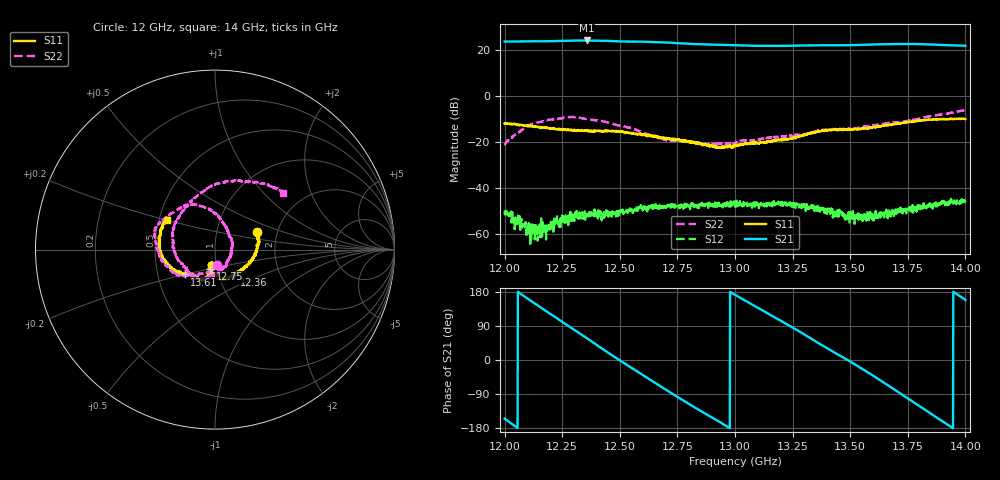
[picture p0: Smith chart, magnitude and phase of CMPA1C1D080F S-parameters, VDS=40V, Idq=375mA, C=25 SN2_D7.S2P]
!Keysight Technologies,E5071C,MY46632380,B.14.03
!Date: Thu Nov 05 05:05:17 2020
!Data & Calibration Information:
!Freq	S11:SOLT2(ON)	S21:SOLT2(ON)	S12:SOLT2(ON)	S22:SOLT2(ON)
!PortZ  Port1:50+j0  Port2:50+j0
!Above PortZ is port z conversion or system Z0 setting when saving the data.
!When reading, reference impedance value at option line is always used.
# Hz S dB R 50
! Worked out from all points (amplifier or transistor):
!   1601 points, 12 GHz to 14 GHz, reference 50 ohm
!   highest |S21| = 24.2 dB at 12.36 GHz (marker M1)
!   |S21| within 3 dB of that: start of sweep to end of sweep
!   unconditionally stable (mu >= 1): start of sweep to end of sweep
!   at 12.33 GHz: K = 11.18, MAG = 24.8 dB, |S12| = -52.4 dB
!   at 13 GHz: K = 8.22, MAG = 22.2 dB, |S12| = -46.5 dB
!   at 14 GHz: K = 5.41, MAG = 23.5 dB, |S12| = -45.8 dB
!   S11 on the Smith chart (normalised r, x): 12 GHz: 1.57, +0.33; 12.36 GHz: 1.19, -0.34; 12.75 GHz: 0.93, -0.20; 13.61 GHz: 0.69, -0.20; 14 GHz: 0.55, +0.20
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1.2e10  -11.89 23.0  23.66 -154.8  -49.85 179.3  -21.33 -83.0
1.206625e10  -12.55 3.3  23.71 176.2  -55.32 -169.0  -15.46 -124.9
1.213625e10  -13.25 -13.9  23.78 147.0  -59.64 -141.7  -11.72 -150.4
1.223625e10  -14.19 -32.4  23.93 106.5  -56.67 -133.8  -9.79 177.0
1.233375e10  -14.94 -46.7  24.13 66.9  -50.95 -144.2  -9.59 150.0
1.235625e10  -14.92 -49.9  24.15 57.8  -51.04 -154.9  -9.87 143.1
1.236375e10  -15.06 -52.1  24.11 54.9  -52.25 -150.7  -10.09 139.6
1.2435e10  -14.97 -63.1  23.97 25.0  -51.33 -164.0  -11.10 115.5
1.250125e10  -15.33 -74.3  23.74 -1.4  -50.03 -156.0  -12.87 98.4
1.258e10  -16.52 -87.3  23.63 -32.0  -48.98 -160.6  -14.91 81.2
1.26675e10  -17.91 -100.2  23.37 -65.9  -47.79 171.1  -17.87 56.0
1.274875e10  -19.07 -104.0  23.01 -96.9  -47.52 157.4  -19.40 31.0
1.28775e10  -21.39 -110.2  22.39 -143.8  -46.92 138.5  -20.95 -5.0
1.3e10  -21.38 -95.5  22.08 172.0  -46.51 113.6  -20.31 -46.9
1.318e10  -19.19 -98.5  21.78 109.8  -46.61 86.0  -17.93 -82.0
1.333375e10  -15.86 -106.5  22.02 55.1  -48.13 51.0  -15.78 -106.2
1.34775e10  -14.34 -129.2  22.06 3.5  -53.57 28.9  -13.92 -139.4
1.361375e10  -13.23 -140.6  22.45 -46.9  -52.81 28.9  -12.69 171.0
1.36675e10  -12.50 -145.8  22.53 -68.2  -49.54 20.3  -11.66 152.6
1.37575e10  -11.23 -161.7  22.63 -104.3  -48.74 11.7  -10.59 119.5
1.38575e10  -10.21 176.8  22.38 -144.5  -48.12 -12.9  -8.52 85.0
1.4e10  -9.97 148.3  21.86 158.7  -45.81 -67.9  -6.14 39.8
